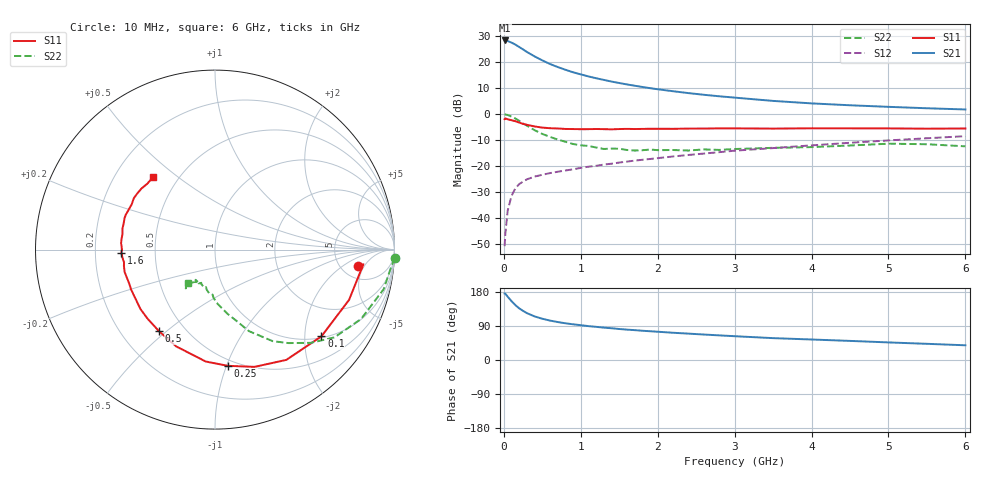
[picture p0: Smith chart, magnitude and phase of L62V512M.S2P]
!  INFINEON TECHNOLOGIES Small Signal Semiconductors
! BFR380L3 , Si-NPN RF-Transistor in TSLP-3-1
!  Vce=2.5 V,  Ic=12.5 mA
! Common Emitter S-Parameters:  07. March 2005
#  GHz  S  MA  R  50
! f  S11  S21  S12  S22
! GHz  Mag  Ang  Mag  Ang  Mag  Ang  Mag  Ang
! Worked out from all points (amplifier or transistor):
!   36 points, 10 MHz to 6 GHz, reference 50 ohm
!   highest |S21| = 28.4 dB at 10 MHz (marker M1)
!   |S21| within 3 dB of that: start of sweep to 225.8 MHz
!   unconditionally stable (mu >= 1): 2.015 GHz to 4.803 GHz
!   at 250 MHz: K = 0.29, MSG = 25.4 dB, |S12| = -25.9 dB
!   at 1.4 GHz: K = 0.92, MSG = 15.8 dB, |S12| = -19.0 dB
!   at 6 GHz: K = 0.97, MSG = 5.1 dB, |S12| = -8.5 dB
!   S11 on the Smith chart (normalised r, x): 10 MHz: 7.21, -3.67; 100 MHz: 1.04, -2.42; 250 MHz: 0.45, -1.01; 500 MHz: 0.36, -0.47; 1.6 GHz: 0.31, -0.02; 6 GHz: 0.36, +0.41
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0.01  0.802 -6.5  26.15 175.5  0.0029 83.5  1.003 -2.7
0.02  0.8308 -5.6  26.02 174.9  0.0051 87.9  0.9867 -5.5
0.05  0.7979 -20.5  25.47 167.0  0.014 79.3  0.9654 -13.2
0.1  0.765 -39.2  23.76 155.3  0.0268 72.0  0.901 -25.4
0.15  0.7318 -57.1  21.78 144.8  0.0376 64.5  0.826 -36.3
0.2  0.6894 -71.4  19.57 136.3  0.0453 59.8  0.7451 -44.2
0.25  0.6515 -83.7  17.57 129.6  0.0507 55.1  0.6628 -51.8
0.3  0.6258 -94.7  15.72 123.7  0.0559 52.7  0.6028 -57.8
0.4  0.581 -111.8  12.9 115.0  0.0632 49.5  0.492 -67.4
0.5  0.5515 -124.4  10.83 108.9  0.0684 48.6  0.4174 -73.0
0.6  0.5379 -134.3  9.221 104.0  0.0737 48.3  0.3664 -78.7
0.7  0.5312 -141.5  8.067 100.2  0.0782 49.3  0.3252 -83.7
0.9  0.5177 -154.6  6.396 94.2  0.0872 50.8  0.2669 -91.9
1.1  0.5153 -162.3  5.323 89.4  0.0978 52.7  0.2457 -97.6
1.4  0.5119 -172.0  4.238 83.8  0.1117 55.1  0.2179 -104.3
1.6  0.5222 -178.0  3.733 80.2  0.1224 56.3  0.2049 -112.0
2.2  0.5226 170.6  2.762 71.9  0.1539 59.2  0.2046 -117.0
2.8  0.5339 160.7  2.21 65.0  0.1861 60.9  0.2057 -124.3
3.5  0.5282 151.6  1.8 57.7  0.2229 60.5  0.2255 -125.3
4.5  0.5344 144.7  1.484 50.4  0.2819 60.6  0.25 -126.5
5.5  0.5264 135.9  1.3 42.7  0.3446 58.2  0.2644 -127.6
6  0.5309 130.5  1.232 38.8  0.378 56.3  0.2409 -129.3
